ORGANIZATION_BLOCK Siemens_AWL1_src
TITLE = Beispiel fuer OB 1 mit unterschiedlichen Bausteinaufrufen
// taken from the Siemens S7 Help/Instruction List examples
// Die 3 dargestellten Netzwerke zeigen Bausteinaufrufe
// mit und ohne Parameter

{S7_pdiag := 'true'} //Systemattribut fuer Bausteine
AUTHOR : Siemens
FAMILY : Beispiel
NAME : Siemens_AWL1_src
VERSION : 1.1
VAR_TEMP
Zwischenwert : INT; // Zwischenspeicher
END_VAR

BEGIN

NETWORK
TITLE = Aufruf einer Funktion mit Uebergabe von Parametern
// Einzeiliger Parameteruebergabe
CALL FC1 (param1 :=E0.0,param2 :=E0.1);


NETWORK
TITLE = Aufruf eines Funktionsbausteins mit
//Uebergabe von Parametern
// Mehrzeilige Parameterangabe
CALL Ampelsteuerung, DB 6 ( // Name des FBs, Instanz-Datenbaustein
dur_g_p := S5T#10S, // Zuweisung aktueller Werte an Parameter

del_r_p := S5T#30S,
starter := TRUE,
t_dur_y_car := T 2,
t_dur_g_ped := T 3,
t_delay_y_car := T 4,
t_dur_r_car := T 5,
t_next_red_car := T 6,
r_car := "re_main", // Anfuehrungszeichen kennzeichnen
y_car := "ye_main", // Namen der Symboltabelle
g_car := "gr_main",
r_ped := "re_int",
g_ped := "gr_int");


NETWORK
TITLE = Aufruf eines Funktionsbausteins mit
//Uebergabe von Parametern
// Einzeilige Parameterangabe
CALL FB10, DB100 (para1 :=E0.0,para2 :=E0.1);

END_ORGANIZATION_BLOCK
